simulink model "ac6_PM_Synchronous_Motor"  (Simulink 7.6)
settings: Solver=FixedStepDiscrete  StartTime=0.0  StopTime=6  FixedStep=Ts  RelTol=1e-3
InitFcn:
  | Ts=1e-5;
  | clc
  | delete *.mat
StartFcn:
  | clc
StopFcn:
  | close all
  | load Csg_Vit.mat
  | plot(x(1,:),x(2,:),x(1,:),x(3,:))
  | title('Consigne vitesse et vitesse de rotation')
  | xlabel('temps')
  | grid
  | 
  | figure
  | load Is_Te.mat
  | plot(y(1,:),y(2,:),y(1,:),y(3,:))
  | title('Courant stator (Phase A) et couple éléctromagnétique')
  | xlabel('temps')
  | grid
libraries: powerlib x2, powerlib_extras x1, electricdrivelib x1

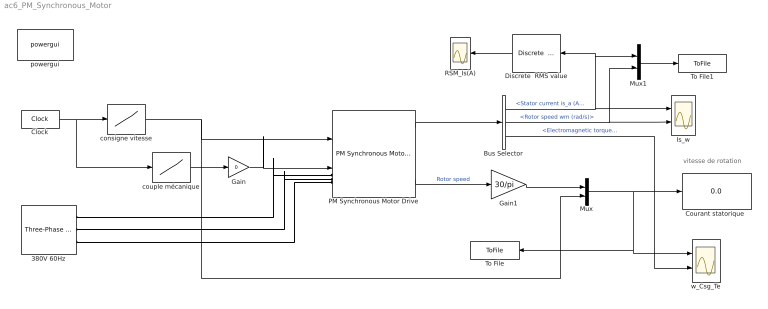
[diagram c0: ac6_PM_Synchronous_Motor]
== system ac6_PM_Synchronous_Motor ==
  note: vitesse de rotation
  380V 60Hz : powerlib/Electrical Sources/Three-Phase Source  DialogController=POWERSYS.PowerSysDialog  SystemSampleTime=-1  Voltage=380  PhaseAngle=0  Frequency=60  InternalConnection=Yg  SpecifyImpedance=off  Resistance=0.02  Inductance=0.05e-3  ShortCircuitLevel=100e6  BaseVoltage=25e3  XRratio=7
  Bus Selector : BusSelector  OutputSignals=Stator current is_a (A),Rotor speed wm (rad/s),Electromagnetic torque Te (N*m)
  Clock : Clock
  "Courant statorique " : Display
  Discrete  RMS value : powerlib_extras/Discrete Measurements/Discrete  RMS value  DialogController=POWERSYS.PowerSysDialog  SystemSampleTime=-1  Freq=60  Mag_Init=0  Ts=Ts
  Gain : Gain  Gain=0
  Gain1 : Gain  Gain=30/pi
  Is_w : Scope  NumInputPorts=2
  Mux : Mux  Inputs=2
  Mux1 : Mux  Inputs=2
  PM Synchronous Motor Drive : electricdrivelib/AC drives/PM Synchronous Motor Drive  SystemSampleTime=-1  showMaskWarnings=on  AverageValue=off  MechanicalLoad=Torque Tm  driveType=AC6
  RSM_Is(A) : Scope
  To File : ToFile  Filename=Csg_Vit  MatrixName=x
  To File1 : ToFile  Filename=Is_Te  MatrixName=y
  consigne vitesse : Lookup  InputValues=[0 0.25 2 4 5 6]  Table=[0 0 200 200 50 50]
  couple mécanique : Lookup  InputValues=[0 0.5 0.501 1.75 1.7501 2.25 2.2501 6]  Table=[0 0 -18 -18 -18 -18 0 0]
  powergui : powerlib/powergui  Priority=2  SystemSampleTime=-1  SimulationMode=Discrete  SampleTime=Ts  frequency=60  SPID=off  DisableSnubberDevices=off  DisableRonSwitches=off  DisableVfSwitches=off  SwTol=0  Interpol=off  frequencyindice=60  echomessages=off  HookPort=off  DisplayEquations=off  FunctionMessages=off  EnableUseOfTLC=off  x0status=blocks  RestoreLinks=warning  ResistiveCurrentMeasurement=off  Frange=[0:2:500]  Ylog=off  Xlog=on  ShowGrid=off  save=off  variable=ZData  ZoomFFT=on  StartTime=0.0  cycles=1  DisplayStyle=1  fundamental=60  FreqAxis=off  MaxFrequency=1000  frequencyindicesteady=1  RmsSteady=1  display=off  Ts=0  methode=off
  w_Csg_Te : Scope  NumInputPorts=2
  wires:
  consigne vitesse/1 -> Mux/2, PM Synchronous Motor Drive/1
  Clock/1 -> consigne vitesse/1, couple mécanique/1
  Mux/1 -> "Courant statorique "/1, w_Csg_Te/1, To File/1
  PM Synchronous Motor Drive/1 -> Bus Selector/1
  Gain1/1 -> Mux/1
  Mux1/1 -> To File1/1
  Bus Selector/1 -> Is_w/1, Mux1/1, Discrete  RMS value/1  "<Stator current is_a (A)>"
  Bus Selector/2 -> Is_w/2, Mux1/2  "<Rotor speed wm (rad/s)>"
  PM Synchronous Motor Drive/4 -> Gain1/1  "Rotor speed"
  couple mécanique/1 -> Gain/1
  Discrete  RMS value/1 -> RSM_Is(A)/1
  Bus Selector/3 -> w_Csg_Te/2  "<Electromagnetic torque Te (N*m)>"
  Gain/1 -> PM Synchronous Motor Drive/2
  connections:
  380V 60Hz/RConn1 -- PM Synchronous Motor Drive/LConn1
  380V 60Hz/RConn2 -- PM Synchronous Motor Drive/LConn2
  380V 60Hz/RConn3 -- PM Synchronous Motor Drive/LConn3
